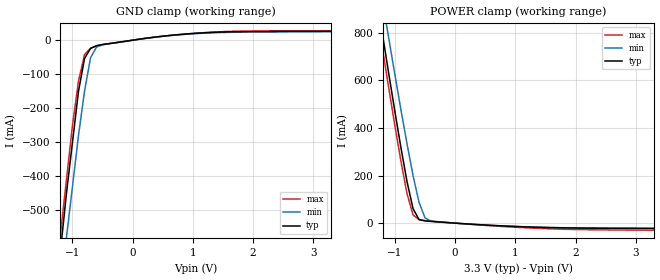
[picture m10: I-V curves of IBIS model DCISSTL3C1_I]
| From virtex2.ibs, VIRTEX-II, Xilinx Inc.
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|   Model DCISSTL3C1_I
[Model]   DCISSTL3C1_I
Model_type   Input
Vinh = 1.7V
Vinl = 1.3V
Polarity   Non-Inverting
C_comp   7.00pF   6.00pF   8.00pF
[Temperature Range]   25.00   100.00   0.000
[Voltage Range]   3.30V   3.00V   3.60V
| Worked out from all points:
|   GND clamp passes 1 mA (typ) near -0.04 V on its own axis
|   POWER clamp passes 1 mA (typ) near -0.06 V on its own axis
[GND_clamp]
| voltage   I(typ)   I(min)   I(max)
-3.3V     -4.3A      -4.31A     -4.26A
-1.2V     -620mA     -740mA     -570mA
-1.1V     -450mA     -580mA     -410mA
-1V       -300mA     -430mA     -250mA
-900mV    -150mA     -280mA     -120mA
-800mV    -54.01mA   -150mA     -42.4mA
-700mV    -24mA      -51.84mA   -23.98mA
-600mV    -16.42mA   -20.12mA   -15.99mA
-500mV    -12.98mA   -13.59mA   -12.47mA
500mV     11.71mA    11.39mA    11.59mA
1.6V      24.44mA    23.02mA    25.9mA
3.3V      26mA       25.18mA    27.78mA
[POWER_clamp]
| voltage   I(typ)   I(min)   I(max)
-3.3V     4.254A     4.222A     4.196A
-1.3V     941.8mA    1.075A     881.3mA
-1.2V     781.2mA    922.7mA    720.7mA
-1.1V     622.4mA    771.2mA    562.1mA
-900mV    315.6mA    475mA      258.2mA
-800mV    174.5mA    333.3mA    123.9mA
-700mV    60.87mA    200.2mA    34.54mA
-600mV    14.89mA    86.98mA    14.92mA
-500mV    9.292mA    21.84mA    10.85mA
-400mV    7.216mA    8.404mA    8.491mA
1.4V      -17.49mA   -17.44mA   -22.15mA
3.3V      -22.37mA   -21.94mA   -29.81mA
